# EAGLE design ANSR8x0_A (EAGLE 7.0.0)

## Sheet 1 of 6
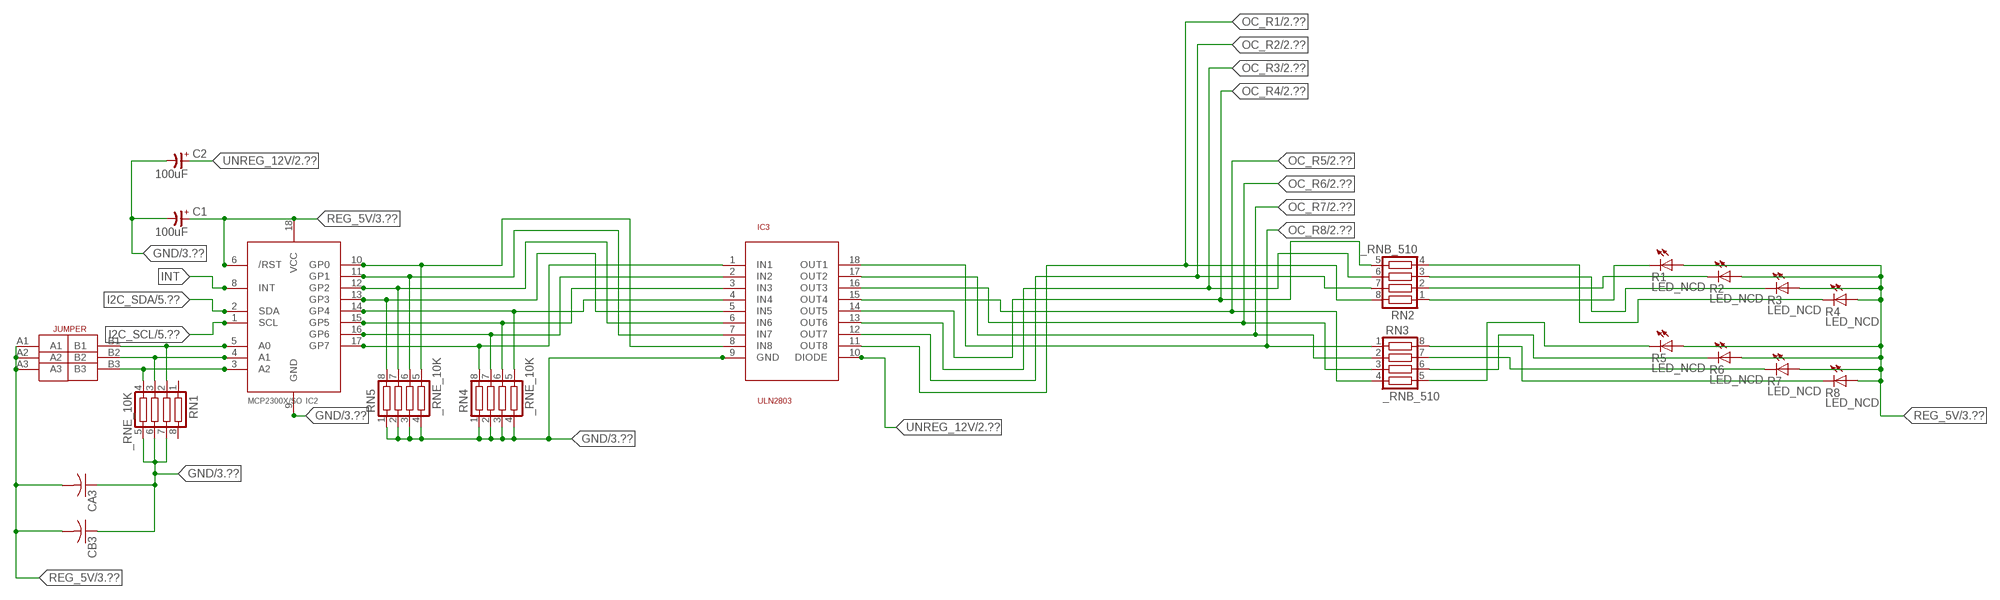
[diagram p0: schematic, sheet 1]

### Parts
C1  100uF  CP-E-025X060  [E-025X060]
C2  100uF  CP-E-025X060  [E-025X060]
CA3  CC1206KRX7R9BB104C1206K  [CC1206KRX7R9BB104]
CB3  TMK316F106ZL-TC1206K  [TMK316F106ZL-T]
IC2  MCP2300X/SO  [SO18W]
IC3  ULN2803  [SO18L]
R1  LED_NCD  [CHIPLED_0603]
R2  LED_NCD  [CHIPLED_0603]
R3  LED_NCD  [CHIPLED_0603]
R4  LED_NCD  [CHIPLED_0603]
R5  LED_NCD  [CHIPLED_0603]
R6  LED_NCD  [CHIPLED_0603]
R7  LED_NCD  [CHIPLED_0603]
R8  LED_NCD  [CHIPLED_0603]
RN1  _RNE_10K  [RNE]
RN2  _RNB_510  [RNB]
RN3  _RNB_510  [RNB]
RN4  _RNE_10K  [RNE]
RN5  _RNE_10K  [RNE]
U$18  JUMPER_3X2  [JUMPER_3X2]

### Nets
GND: C1.- C2.- CA3.1 CB3.1 IC2.9(GND) IC3.9(GND) RN1.5 RN1.6 RN1.7 RN4.1 RN4.2 RN4.3 RN4.4 RN5.1 RN5.2 RN5.3 RN5.4 ; also sheet 3,4,5,6
GP4: IC2.14(GP4) IC3.4(IN4) RN4.5
GP6: IC2.16(GP6) IC3.2(IN2) RN4.7
I2C_SCL: IC2.1(SCL) ; also sheet 5,6
I2C_SDA: IC2.2(SDA) ; also sheet 5,6
INT: IC2.8(INT)
N$6: IC2.5(A0) RN1.2 U$18.B1
N$7: IC2.4(A1) RN1.3 U$18.B2
N$8: IC2.3(A2) RN1.4 U$18.B3
N$20: R1.C RN2.1
N$21: IC2.12(GP2) IC3.6(IN6) RN5.7
N$22: IC2.11(GP1) IC3.7(IN7) RN5.6
N$23: IC2.10(GP0) IC3.8(IN8) RN5.5
N$29: R2.C RN2.2
N$30: R3.C RN2.3
N$31: R4.C RN2.4
N$32: R8.C RN3.8
N$81: R7.C RN3.7
N$82: R6.C RN3.6
N$83: R5.C RN3.5
N$89: IC2.13(GP3) IC3.5(IN5) RN5.8
N$93: IC2.15(GP5) IC3.3(IN3) RN4.6
N$94: IC2.17(GP7) IC3.1(IN1) RN4.8
OC_R1: IC3.11(OUT8) RN2.8 ; also sheet 2
OC_R2: IC3.12(OUT7) RN2.7 ; also sheet 2
OC_R3: IC3.13(OUT6) RN2.6 ; also sheet 2
OC_R4: IC3.14(OUT5) RN2.5 ; also sheet 2
OC_R5: IC3.15(OUT4) RN3.4 ; also sheet 2
OC_R6: IC3.16(OUT3) RN3.3 ; also sheet 2
OC_R7: IC3.17(OUT2) RN3.2 ; also sheet 2
OC_R8: IC3.18(OUT1) RN3.1 ; also sheet 2
REG_5V: C1.+ CA3.2 CB3.2 IC2.6(/RST) IC2.18(VCC) R1.A R2.A R3.A R4.A R5.A R6.A R7.A R8.A U$18.A1 U$18.A2 U$18.A3 ; also sheet 3,4,5,6
UNREG_12V: C2.+ IC3.10(DIODE) ; also sheet 2,3
Unconnected: RN1.1 RN1.8

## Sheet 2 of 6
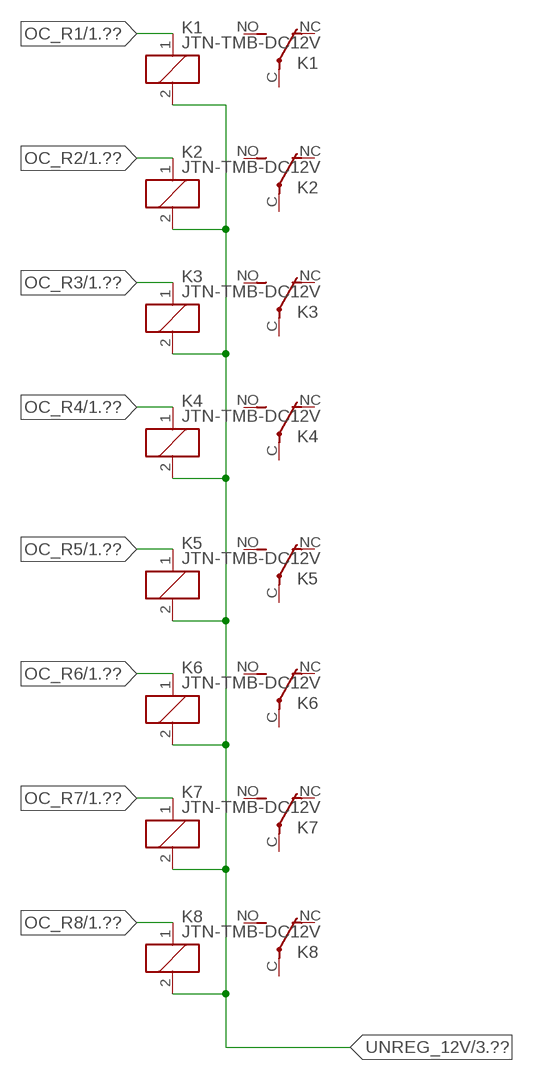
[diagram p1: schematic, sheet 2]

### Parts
K1  JTN-TMB-DC12V  [JT-TMB]
K2  JTN-TMB-DC12V  [JT-TMB]
K3  JTN-TMB-DC12V  [JT-TMB]
K4  JTN-TMB-DC12V  [JT-TMB]
K5  JTN-TMB-DC12V  [JT-TMB]
K6  JTN-TMB-DC12V  [JT-TMB]
K7  JTN-TMB-DC12V  [JT-TMB]
K8  JTN-TMB-DC12V  [JT-TMB]

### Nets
OC_R1: K1.1(C1) ; also sheet 1
OC_R2: K2.1(C1) ; also sheet 1
OC_R3: K3.1(C1) ; also sheet 1
OC_R4: K4.1(C1) ; also sheet 1
OC_R5: K5.1(C1) ; also sheet 1
OC_R6: K6.1(C1) ; also sheet 1
OC_R7: K7.1(C1) ; also sheet 1
OC_R8: K8.1(C1) ; also sheet 1
UNREG_12V: K1.2(C2) K2.2(C2) K3.2(C2) K4.2(C2) K5.2(C2) K6.2(C2) K7.2(C2) K8.2(C2) ; also sheet 1,3
Unconnected: K1.C(COM) K1.NC K1.NO K2.C(COM) K2.NC K2.NO K3.C(COM) K3.NC K3.NO K4.C(COM) K4.NC K4.NO K5.C(COM) K5.NC K5.NO K6.C(COM) K6.NC K6.NO K7.C(COM) K7.NC K7.NO K8.C(COM) K8.NC K8.NO

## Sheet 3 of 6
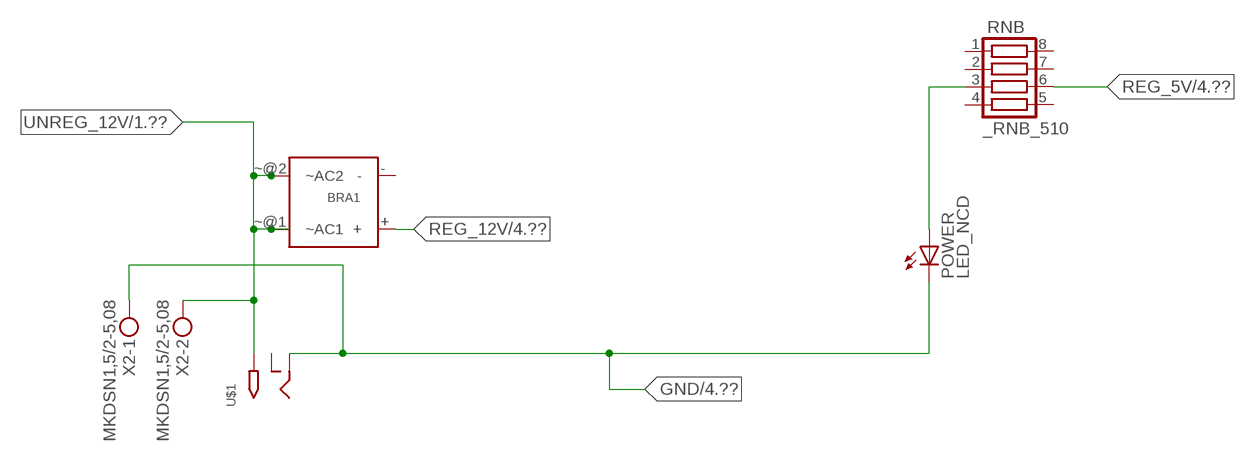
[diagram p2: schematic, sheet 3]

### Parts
BRA1  MB2S_  [MB2S]
POWER  LED_NCD  [CHIPLED_0603]
RNB  _RNB_510  [RNB]
U$1  2.1MMJACK  [PJ-102A]
X2  MKDSN1,5/2-5,08  [MKDSN1,5/2-5,08]

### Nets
GND: POWER.C U$1.RING X2.1 ; also sheet 1,4,5,6
N$2: POWER.A RNB.3
REG_5V: RNB.6 ; also sheet 1,4,5,6
REG_12V: BRA1.+ ; also sheet 4
UNREG_12V: BRA1.~@1(~AC1) BRA1.~@2(~AC2) U$1.TIP X2.2 ; also sheet 1,2
Unconnected: BRA1.- RNB.1 RNB.2 RNB.4 RNB.5 RNB.7 RNB.8 U$1.RING_SW

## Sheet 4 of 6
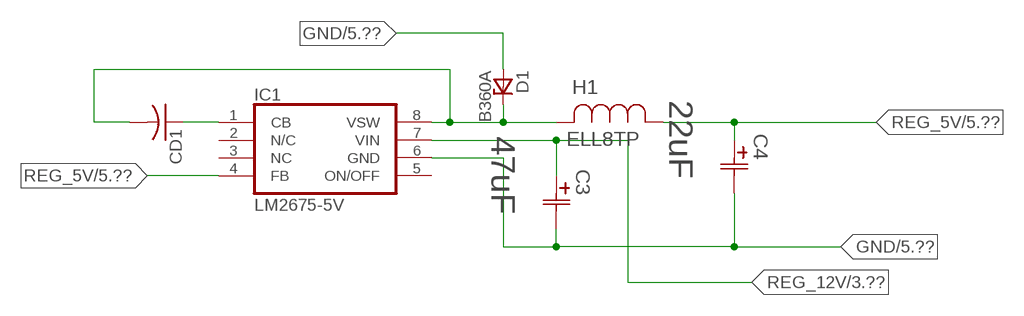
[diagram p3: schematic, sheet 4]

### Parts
C3  47uF  490-5463-6-NDCAP  [C2917(7343)-Y]
C4  22uF  490-5463-6-NDCAP  [C2917(7343)-Y]
CD1  _CD_10NF_50VC1206K  [_CD_10NF_50V]
D1  B360A  [DO214AC_ZENER]
H1  ELL8TP  [IND_ELL8TP]
IC1  LM2675-5V  LM2675  [SO-8]

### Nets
GND: C3.2(C2) C4.2(C2) D1.A IC1.6(GND) ; also sheet 1,3,5,6
N$1: CD1.2 D1.C H1.2 IC1.8(VSW)
N$3: CD1.1 IC1.1(CB)
REG_5V: C4.1(C1) H1.1 IC1.4(FB) ; also sheet 1,3,5,6
REG_12V: C3.1(C1) IC1.7(VIN) ; also sheet 3
Unconnected: IC1.2(N/C) IC1.5(ON/OFF)

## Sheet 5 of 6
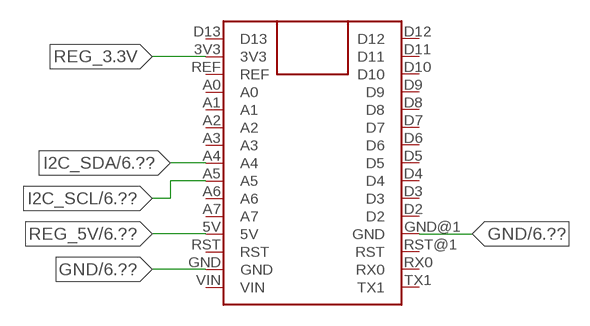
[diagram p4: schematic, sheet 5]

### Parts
FOR_NANO  ARDUINO_NANO  [ARDUINO_NANO]

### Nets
GND: FOR_NANO.GND FOR_NANO.GND@1(GND) ; also sheet 1,3,4,6
I2C_SCL: FOR_NANO.A5 ; also sheet 1,6
I2C_SDA: FOR_NANO.A4 ; also sheet 1,6
REG_3.3V: FOR_NANO.3V3
REG_5V: FOR_NANO.5V ; also sheet 1,3,4,6
Unconnected: FOR_NANO.A0 FOR_NANO.A1 FOR_NANO.A2 FOR_NANO.A3 FOR_NANO.A6 FOR_NANO.A7 FOR_NANO.D2 FOR_NANO.D3 FOR_NANO.D4 FOR_NANO.D5 FOR_NANO.D6 FOR_NANO.D7 FOR_NANO.D8 FOR_NANO.D9 FOR_NANO.D10 FOR_NANO.D11 FOR_NANO.D12 FOR_NANO.D13 FOR_NANO.REF FOR_NANO.RST FOR_NANO.RST@1(RST) FOR_NANO.RX0 FOR_NANO.TX1 FOR_NANO.VIN

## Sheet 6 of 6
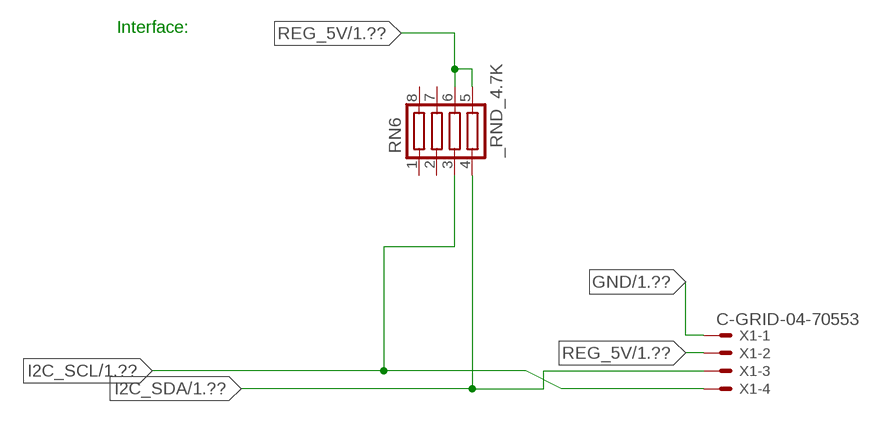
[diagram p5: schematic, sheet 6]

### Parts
RN6  _RND_4.7K  [RND]
X1  C-GRID-04-70553  [70553-04]

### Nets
GND: X1.1 ; also sheet 1,3,4,5
I2C_SCL: RN6.3 X1.4 ; also sheet 1,5
I2C_SDA: RN6.4 X1.3 ; also sheet 1,5
REG_5V: RN6.5 RN6.6 X1.2 ; also sheet 1,3,4,5
Unconnected: RN6.1 RN6.2 RN6.7 RN6.8

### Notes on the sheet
- Interface:

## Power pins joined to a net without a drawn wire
NC: IC1.3(NC)

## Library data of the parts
BRA1 = NCD_ULTIMATE_LIBRARY:MB2S: Bridge Rectifier BRA MB2S 200V 500ma Digikey MB2S-TPMSTR-ND/MB2S-TP
C1 C2 = NCD_ULTIMATE_LIBRARY:CP-: Capacitors All Kinds POLARIZED CAP
C3 C4 = NCD_ULTIMATE_bhaskar:490-5463-6-ND: NCD CAP
CA3 = NCD_ULTIMATE_LIBRARY:CC1206KRX7R9BB104: Capacitor CA .1uF 50V SMT C1206K CC1206KRX7R9BB104
CB3 = NCD_ULTIMATE_LIBRARY:TMK316F106ZL-T: Capacitor CB 10uF SMT 1206 TMK316F106ZL-T
CD1 = NCD_ULTIMATE_LIBRARY:_CD_10NF_50V: Capacitor 10nF SMT
D1 = NCD_ULTIMATE_bhaskar:B360A: NCD DIODE B350A/B360A
FOR_NANO = NCD_ULTIMATE_CONNECTORS:ARDUINO_NANO
H1 = NCD_ULTIMATE_bhaskar:ELL8TP: NCD coil
IC1 = NCD_ULTIMATE_bhaskar:LM2675: LM2675 NCD http://www.ti.com/lit/ds/symlink/lm2675.pdf
IC2 = NCD_ULTIMATE_LIBRARY:MCP2300X: Semiconductor Port Expander I/O 8-Bit I2C MCP23008 Inexpensive i2c i/o expander - 8 general purpose i/o pins with optional pullups
IC3 = NCD_ULTIMATE_LIBRARY:ULN2803: Semiconductor 8 O.C. N-Channel Transistor Driver Digikey ULN2803AFWGCELTR-ND/ULN2803AFWG,C,EL
K1-K8 = NCD_ULTIMATE_LIBRARY:JT?-*: RELAY COMPACT ECONOMICAL 30 AMP. RELAY NAiS Source: http://www.mew-europe.com/.. en_ds_61212_0000.pdf
POWER = NCD_ULTIMATE_bhaskar:LED_NCD
R1-R8 = NCD_ULTIMATE_LIBRARY:LED_NCD: LED Digikey 754-1132-2-ND/APT2012SRCPRV
RN1 RN4 RN5 = NCD_ULTIMATE_LIBRARY:_RNE_10K: Resistor Array RNE SMT 10K x 4 Single Resistor Source: http://www.ctscorp.com/components/Datasheets/CTSChipArrayDs.pdf Digikey 742C083103JPTR-ND/742C083103JP; OC_FARNELL: unknown; OC_NEWARK: unknown
RN2 RN3 RNB = NCD_ULTIMATE_LIBRARY:_RNB_510: Resistor Array RNB SMT 510 x 4 Single Resistor Source: http://www.ctscorp.com/components/Datasheets/CTSChipArrayDs.pdf Digikey 742C083511JPTR-ND/ 742C083511JP; OC_FARNELL: unknown; OC_NEWARK: unknown
RN6 = NCD_ULTIMATE_LIBRARY:_RND_4.7K: Resistor Array RND SMT 4.7K x 4 Single Resistor Source: http://www.ctscorp.com/components/Datasheets/CTSChipArrayDs.pdf Digikey 742C083472JPTR-ND/742C083472JP; OC_FARNELL: unknown; OC_NEWARK: unknown
U$1 = NCD_ULTIMATE_CONNECTORS:2.1MMJACK: 2.1mm x 5.5mm DC jack with internal switch. Digikey part #PJ-102A, 4UCON part #05537 By microbuilder.eu
U$18 = NCD_ULTIMATE_CONNECTORS:JUMPER_3X2
X1 = NCD_ULTIMATE_CONNECTORS:C-GRID-04: CONNECTOR 4-Pos I2C wire to board 2.54 mm (0.100") pitch header Digikey WM1342-ND/0015912045; OC_FARNELL: unknown; OC_NEWARK: unknown
X2 = NCD_ULTIMATE_CONNECTORS:MKDSN1,5/2-5,08: MKDSN 1,5/ 2-5,08 Printklemme

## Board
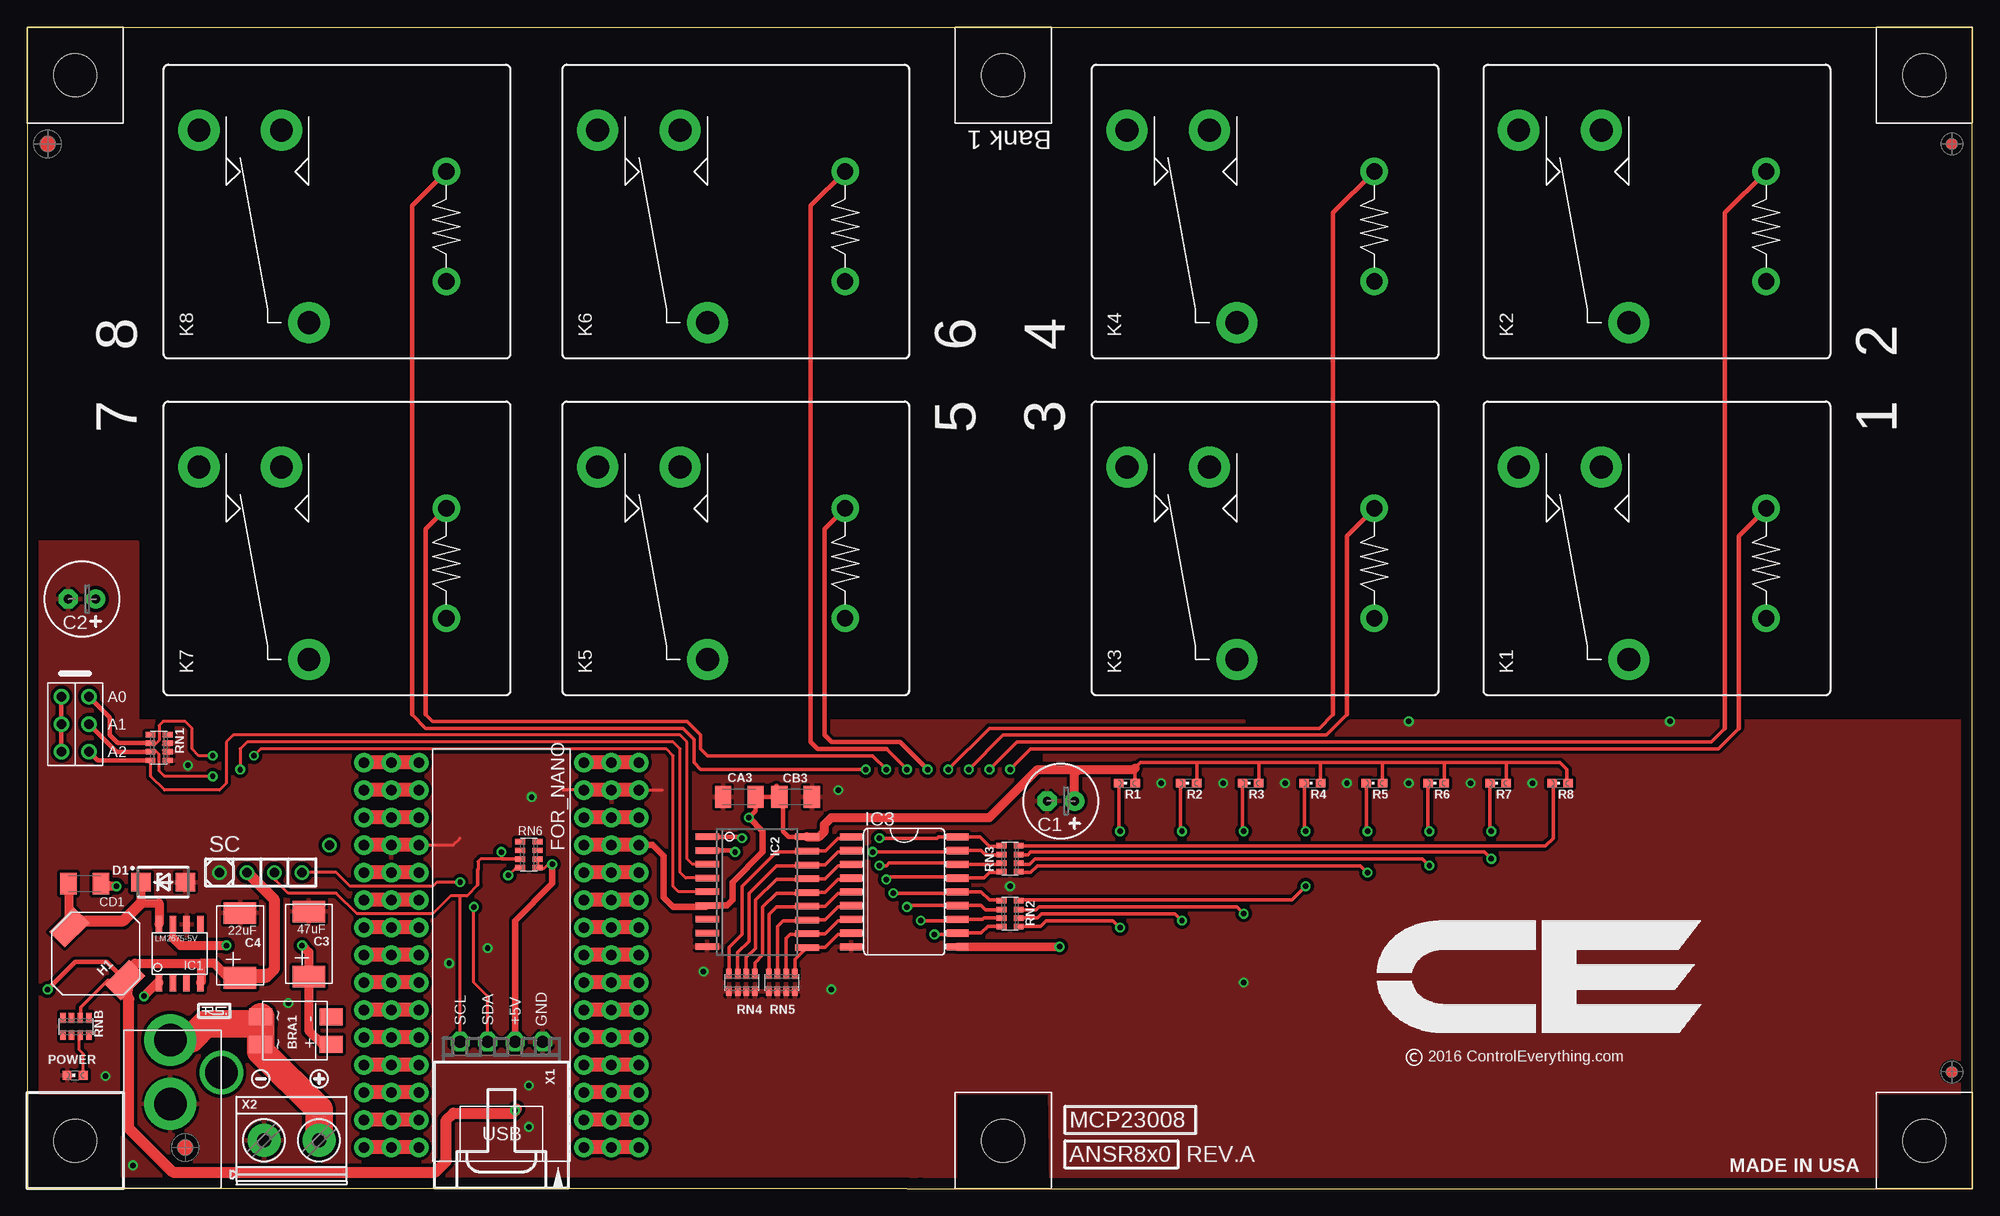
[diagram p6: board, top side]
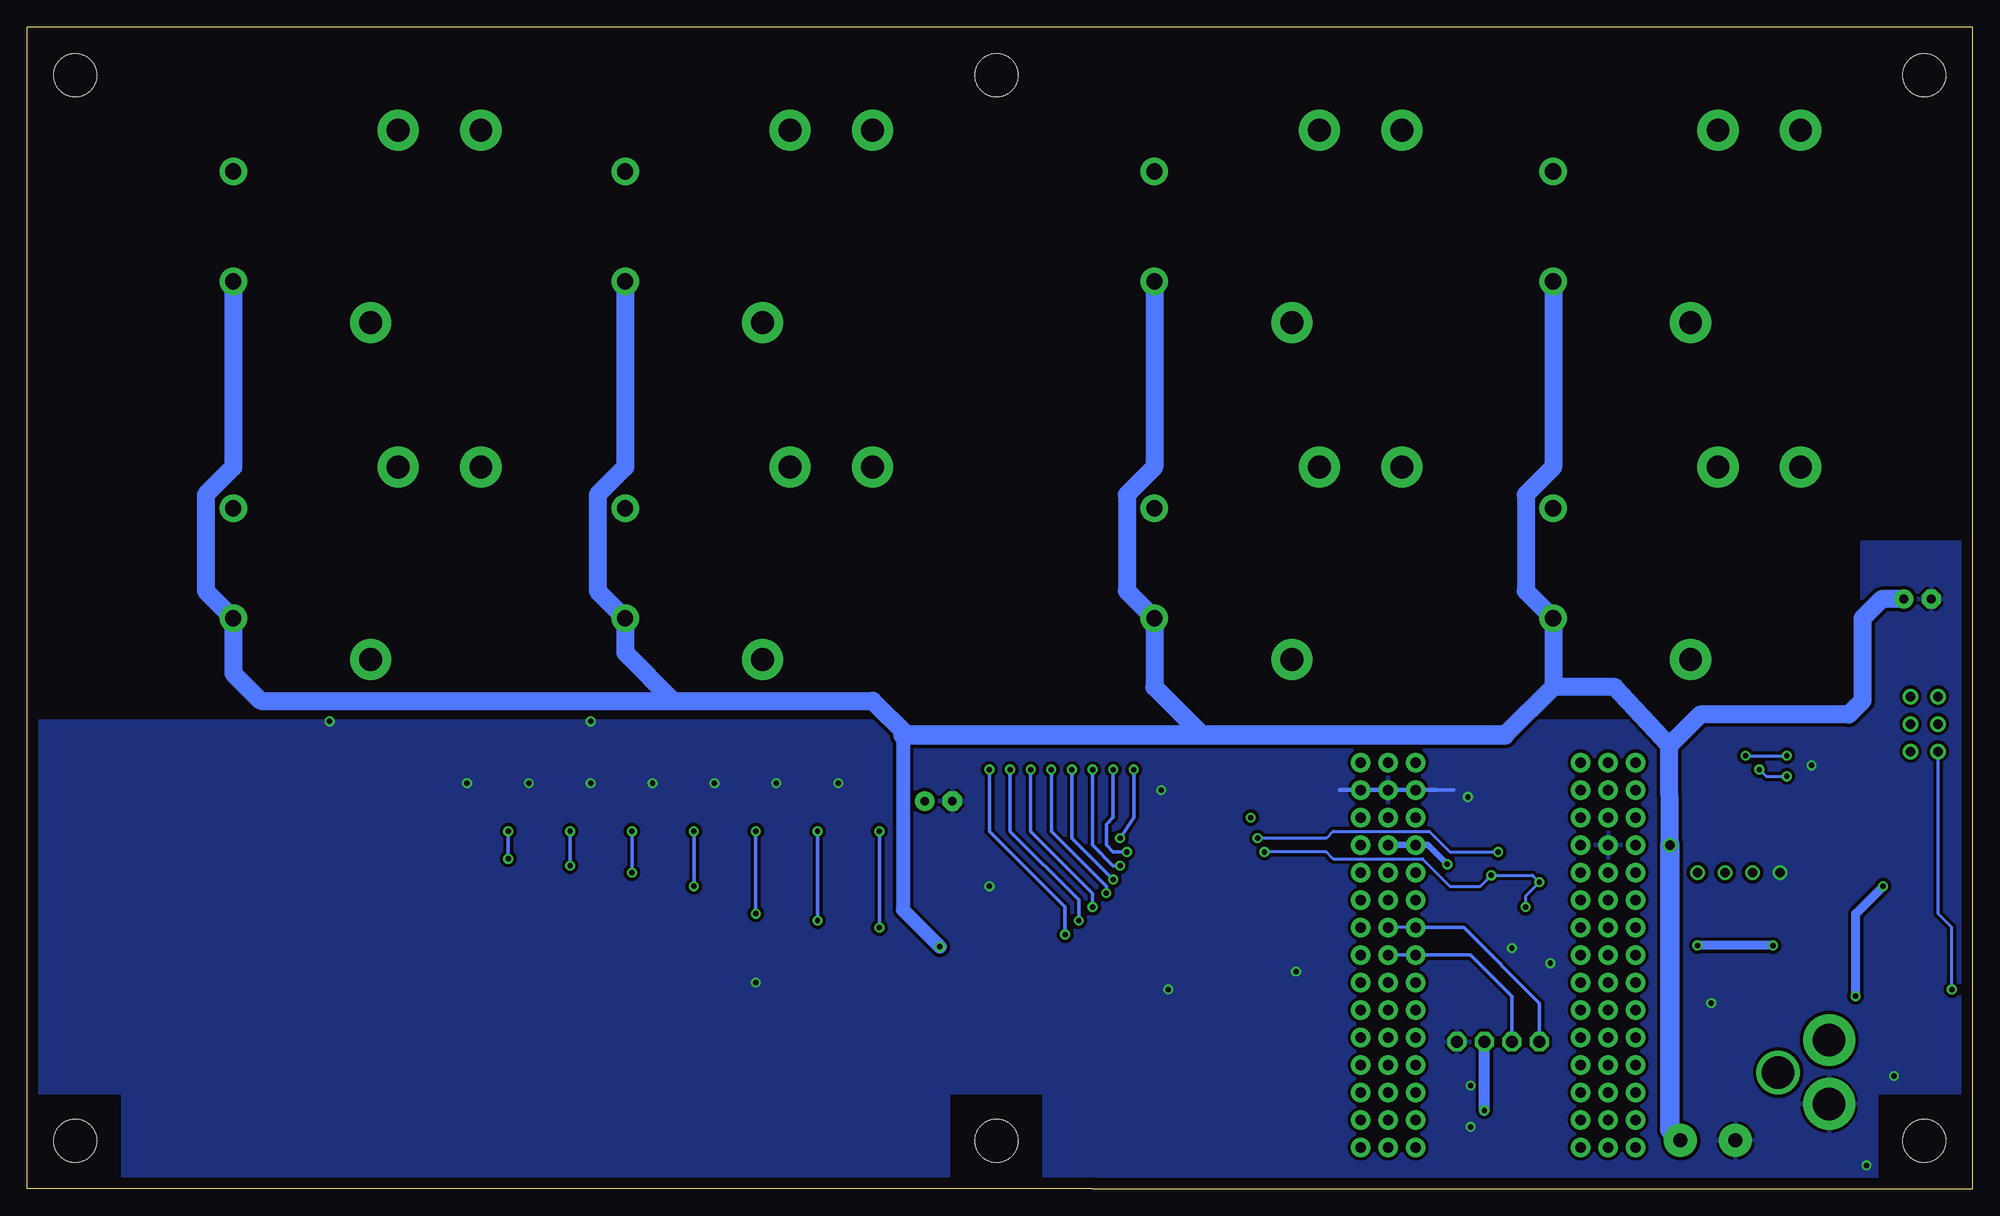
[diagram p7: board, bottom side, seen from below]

Size 179.71 x 107.33 mm. Coordinates in mm from the lower left corner, seen from the top.
Outline: 81.28,0 82.53,0
Outline: 0,65.71 0,64.77
Outline: 0,64.77 0,0 81.28,0
Outline: 81.28,0 179.71,0 179.71,107.31
Outline: 0,107.31 0,64.77
Outline: 0.02,107.33 179.71,107.33
Copper layers (1*16): Top 0.035mm / dielectric 1.5mm / Bottom 0.035mm
Design rules "default": minimum track width 10mil, minimum drill 24mil, track to track 8mil, track to pad 8mil, pad to pad 8mil, via to via 8mil, smd to smd 8mil, copper to edge 40mil, drill to drill 8mil, minimum pad ring 10mil, minimum via ring 8mil, stop-mask expansion 4mil, vias tented up to drill 0mil, thermal gap 10mil
Holes 3.96 mm at 4.45,4.45 4.45,4.45 4.45,4.45 4.45,4.45

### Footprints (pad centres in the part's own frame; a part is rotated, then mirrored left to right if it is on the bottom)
MB2S = smd 1.55 x 2.1: + 0,-6.5; - 2.54,-6.5; ~@1 0,0; ~@2 2.54,0
E-025X060 = drill 0.813 pad 1.778: + -1.27,0 | drill 0.813 pad 1.778 octagon: - 1.27,0
C2917(7343)-Y = smd 2 x 3: 1 -3,0; 2 3,0
CC1206KRX7R9BB104 = smd 1.5 x 2: 1 -1.5,0; 2 1.5,0
TMK316F106ZL-T = smd 1.5 x 2: 1 -1.5,0; 2 1.5,0
_CD_10NF_50V = smd 1.5 x 2: 1 -1.5,0; 2 1.5,0
DO214AC_ZENER = smd 1.8 x 1.7: A 2.05,0; C -2.05,0
ARDUINO_NANO = drill 1 pad 1.778: 3V1 -2.54,-2.54; 3V3 0,-2.54; 5V 0,-27.94; 5V1 -2.54,-27.94; A0 0,-7.62; A1 0,-10.16; A2 0,-12.7; A3 0,-15.24; A4 0,-17.78; A5 0,-20.32; A6 0,-22.86; A7 0,-25.4; A8 -2.54,-7.62; A9 -2.54,-10.16; A10 -2.54,-12.7; A11 -2.54,-15.24; A12 -2.54,-17.78; A13 -2.54,-20.32; A14 -2.54,-22.86; A15 -2.54,-25.4; D1 -2.54,0; D2 20.32,-25.4; D3 20.32,-22.86; D4 20.32,-20.32; D5 20.32,-17.78; D6 20.32,-15.24; D7 20.32,-12.7; D8 20.32,-10.16; D9 20.32,-7.62; D10 20.32,-5.08; D11 20.32,-2.54; D12 20.32,0; D13 0,0; D14 22.86,0; D15 22.86,-2.54; D16 22.86,-5.08; D17 22.86,-7.62; D18 22.86,-10.16; D19 22.86,-12.7; D20 22.86,-15.24; D21 22.86,-17.78; D22 22.86,-20.32; D23 22.86,-22.86; D24 22.86,-25.4; GND 0,-33.02; GND1 -2.54,-33.02; GND@1 20.32,-27.94; GND@2 22.86,-27.94; P$16 2.54,0; P$17 2.54,-2.54; P$18 2.54,-5.08; P$19 2.54,-7.62; P$20 2.54,-10.16; P$21 2.54,-12.7; P$22 2.54,-15.24; P$23 2.54,-17.78; P$24 2.54,-20.32; P$25 2.54,-22.86; P$26 2.54,-25.4; P$27 2.54,-27.94; P$28 2.54,-30.48; P$29 2.54,-33.02; P$30 2.54,-35.56; P$31 17.78,0; P$32 17.78,-2.54; P$33 17.78,-5.08; P$34 17.78,-7.62; P$35 17.78,-10.16; P$36 17.78,-12.7; P$37 17.78,-15.24; P$38 17.78,-17.78; P$39 17.78,-20.32; P$40 17.78,-22.86; P$41 17.78,-25.4; P$42 17.78,-27.94; P$43 17.78,-30.48; P$44 17.78,-33.02; P$45 17.78,-35.56; REF 0,-5.08; REF1 -2.54,-5.08; RST 0,-30.48; RST1 -2.54,-30.48; RST@1 20.32,-30.48; RST@2 22.86,-30.48; RX0 20.32,-33.02; RX1 22.86,-33.02; TX1 20.32,-35.56; TX2 22.86,-35.56; VIN 0,-35.56; VIN1 -2.54,-35.56
IND_ELL8TP = smd 2.054 x 3.2 rotated 45: 1 -2.442,-2.696; 2 2.442,2.442
SO-8 = smd 0.6 x 1.55: 1 -1.905,-2.69; 2 -0.635,-2.69; 3 0.635,-2.69; 4 1.905,-2.69; 5 1.905,2.71; 6 0.635,2.71; 7 -0.635,2.71; 8 -1.905,2.71
SO18W = smd 0.6 x 2.2: 1 -4.445,-4.6; 2 -3.175,-4.6; 3 -1.905,-4.6; 4 -0.635,-4.6; 5 0.635,-4.6; 6 1.905,-4.6; 7 3.175,-4.6; 8 4.445,-4.6; 9 5.715,-4.6; 10 5.775,4.6; 11 4.505,4.6; 12 3.235,4.6; 13 1.965,4.6; 14 0.695,4.6; 15 -0.575,4.6; 16 -1.845,4.6; 17 -3.145,4.6; 18 -4.445,4.6
SO18L = smd 0.66 x 2.032: 1 -5.08,-4.902; 2 -3.81,-4.902; 3 -2.54,-4.902; 4 -1.27,-4.902; 5 0,-4.902; 6 1.27,-4.902; 7 2.54,-4.902; 8 3.81,-4.902; 9 5.08,-4.902; 10 5.08,4.902; 11 3.81,4.902; 12 2.54,4.902; 13 1.27,4.902; 14 0,4.902; 15 -1.27,4.902; 16 -2.54,4.902; 17 -3.81,4.902; 18 -5.08,4.902
JT-TMB = drill 1.5 pad 2.54: 1 5.08,0; 2 -5.08,0 | drill 2.1 pad 3.81: C -8.89,12.7; NC 8.89,22.86; NO 8.89,15.24
CHIPLED_0603 = smd 0.8 x 0.8: A 0,-0.75; C 0,0.75
CHIPLED_0603' = smd 0.8 x 0.876: A 0,-0.75; C 0,0.75
RNE = smd 0.5 x 0.9: 1 -1.2,-0.8; 2 -0.4,-0.8; 3 0.4,-0.8; 4 1.2,-0.8; 5 1.2,0.8; 6 0.4,0.8; 7 -0.4,0.8; 8 -1.2,0.8
RNB = smd 0.5 x 0.9: 1 -1.2,-0.8; 2 -0.4,-0.8; 3 0.4,-0.8; 4 1.2,-0.8; 5 1.2,0.8; 6 0.4,0.8; 7 -0.4,0.8; 8 -1.2,0.8
RND = smd 0.5 x 0.9: 1 -1.2,-0.8; 2 -0.4,-0.8; 3 0.4,-0.8; 4 1.2,-0.8; 5 1.2,0.8; 6 0.4,0.8; 7 -0.4,0.8; 8 -1.2,0.8
PJ-102A = drill 3 pad 4.8: RING 0.1,-3.39; TIP 0.1,-9.29 | drill 3 pad 3.251: RING_SW -4.6,-6.29
PCB_MOUNTING_HOLE = hole 3.962: 4.445,4.445
JUMPER_3X2 = drill 0.9: A1 0,5.08; A2 0,2.54; A3 0,0; B1 2.54,5.08; B2 2.54,2.54; B3 2.54,0
70553-04 = drill 1.1 pad 1.778 octagon: 1 -3.81,-7.62; 2 -1.27,-7.62; 3 1.27,-7.62; 4 3.81,-7.62
MKDSN1,5/2-5,08 = drill 1.3 pad 3.048: 1 -2.561,0.025; 2 2.519,0.025

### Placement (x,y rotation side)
BRA1  21.59,13.34 90 top
C1  95.5,35.81 180 top
C2  5.08,54.48 180 top
C3  26.04,22.61 90 top
C4  19.68,22.48 90 top
CA3  65.79,36.2 0 top
CB3  70.99,36.2 180 top
CD1  5.33,28.19 180 top
D1  12.57,28.32 0 top
FOR_NANO  53.98,3.81 180 top
H1  6.35,21.72 90 top
IC1  14.1,21.72 0 top
IC2  67.44,28.07 270 top
IC3  81.03,27.43 270 top
K1  160.66,57.79 90 top
K2  160.66,88.9 90 top
K3  124.46,57.79 90 top
K4  124.46,88.9 90 top
K5  75.56,57.79 90 top
K6  75.56,88.9 90 top
K7  38.73,57.79 90 top
K8  38.73,88.9 90 top
POWER  4.45,10.48 90 top
R1  LED_NCD  [CHIPLED_0603']  101.6,37.47 90 top
R2  LED_NCD  [CHIPLED_0603']  107.31,37.47 90 top
R3  LED_NCD  [CHIPLED_0603']  113.03,37.47 90 top
R4  LED_NCD  [CHIPLED_0603']  118.75,37.47 90 top
R5  LED_NCD  [CHIPLED_0603']  124.46,37.47 90 top
R6  LED_NCD  [CHIPLED_0603']  130.18,37.47 90 top
R7  LED_NCD  [CHIPLED_0603']  135.89,37.47 90 top
R8  LED_NCD  [CHIPLED_0603']  141.6,37.47 90 top
RN1  12.19,40.77 270 top
RN2  90.81,25.4 90 top
RN3  90.81,30.48 270 top
RN4  66.04,19.05 0 top
RN5  69.72,19.05 0 top
RN6  46.35,30.86 270 top
RNB  4.51,14.99 0 top
U$1  13.34,4.45 180 top
U$2  [VISION_REF15]  14.61,3.81 0 top
U$3  [ICON_MINUS]  21.59,10.16 180 top
U$4  [VISION_REF10]  177.8,10.79 270 top
U$5  [ICON_PLUS]  26.99,10.16 90 top
U$6  PCB_MOUNTING_HOLE  [PCB_MOUNTING_HOLE]  94.61,0 90 top
U$11  PCB_MOUNTING_HOLE  [PCB_MOUNTING_HOLE]  179.71,0 90 top
U$13  [VISION_REF10]  177.8,96.52 270 top
U$14  [VISION_REF15]  1.91,96.52 270 top
U$17  PCB_MOUNTING_HOLE  [PCB_MOUNTING_HOLE]  94.61,98.42 90 top
U$18  3.17,40.39 0 top
U$19  PCB_MOUNTING_HOLE  [PCB_MOUNTING_HOLE]  94.61,98.42 90 top
U$20  PCB_MOUNTING_HOLE  [PCB_MOUNTING_HOLE]  179.71,98.42 90 top
U$21  [ICON_USA]  157.23,1.52 0 top
U$25  PCB_MOUNTING_HOLE  [PCB_MOUNTING_HOLE]  179.71,98.42 90 top
U$31  PCB_MOUNTING_HOLE  [PCB_MOUNTING_HOLE]  8.89,98.42 90 top
U$32  PCB_MOUNTING_HOLE  [PCB_MOUNTING_HOLE]  8.89,98.42 90 top
X1  43.81,5.97 180 top
X2  24.45,4.45 0 top

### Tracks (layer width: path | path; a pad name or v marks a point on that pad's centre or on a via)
GND  (via drill 0.5, 0.9)
  Top 0.254: 36.2,31.75 39.37,31.75 40.01,32.39 | FOR_NANO.GND@1 32.38,31.75 | 49.53,36.83 56.52,36.83 58.67,36.83
  Top 1.016: X1.1 47.62,13.74
  Bottom 0.254: 51.44,36.83 FOR_NANO.GND
  Bottom 0.305: 47.88,36.83 49.53,36.83 51.44,36.83
  Bottom 0.406: 49.53,36.83 58.42,36.83
  other vias: 14.86,39.12 62.48,20.07 127.64,37.47 112.39,19.05 133.35,37.47 139.06,37.47 121.92,37.47 116.2,37.47 110.49,37.47 104.78,37.47 90.81,27.94 127.64,43.18 151.76,43.18 74.3,18.41 74.93,36.83 9.78,2.16 17.78,29.21 46.35,9.53 46.61,36.2 46.35,5.72 42.55,22.23 38.99,20.83 7.24,10.41 24.13,17.15
  pour Bottom (isolate 0.305): -3.17,8.89 8.89,8.89 8.89,0 85.72,0 85.72,8.89 112.39,8.89 112.39,43.18 10.16,43.18 10.16,59.69 -3.17,59.69
  pour Top (isolate 0.305): -1.27,8.89 8.89,8.89 8.89,0 85.72,0 85.72,8.89 112.39,8.89 112.39,43.18 10.16,43.18 10.16,59.69 -1.27,59.69
  pour Top (isolate 0.305): 112.39,43.18 180.97,43.18 181.61,8.89 170.81,8.89 170.81,0 111.76,0
  pour Bottom (isolate 0.305): 94.61,0 94.61,43.18 182.25,43.18 182.88,8.89 170.81,8.89 170.81,0
  pour Top (isolate 0.305): 185.42,8.89 170.81,8.89 170.81,0 94.61,0 93.98,43.18 184.78,43.18
  pour Top (isolate 0.305): 170.81,8.89 170.81,0 94.61,0 93.98,43.18 186.69,43.18 187.32,8.89
GP4
  Top 0.305: RN4.5 67.24,20.88 67.94,21.59 67.94,26.04 69.22,27.3 71.97,27.3 IC2.14 73.73,27.37 74.93,28.57 76,28.57 IC3.4
GP6
  Top 0.305: RN4.7 65.64,21.83 66.67,22.86 66.67,27.3 69.22,29.84 71.97,29.84 IC2.16 73.73,29.91 74.93,31.12 76,31.12 IC3.2
I2C_SCL  (via drill 0.5, 0.9)
  Top 0.254: 41.64,28.05 40.64,27.05 40.01,27.05 | 40.01,27.05 39.12,27.05 37.47,25.4 30.48,25.4 28.57,27.3 24.13,27.3 22.86,28.57 v22.86,29.21 | X1.4 40.01,27.05 | v43.81,31.12 43.81,30.48 45.54,30.48 RN6.3 41.89,30.46 41.66,30.23 41.66,29.5
  Top 0.305: 41.64,28.05 41.64,29.48 41.66,29.5
  Top 0.406: IC2.1 65.91,32.51 v66.04,32.39
  Bottom 0.254: v43.81,31.12 48.26,31.12 50.16,33.02 59.05,33.02 59.69,32.39 v66.04,32.39 | 51.44,24.13 FOR_NANO.A5
  Bottom 0.305: 51.44,24.13 46.99,24.13 40.01,17.15 X1.4
I2C_SDA  (via drill 0.5, 0.9)
  Top 0.254: RN6.4 45.16,29.66 v44.45,28.96 | 40,28.33 v40.01,28.32 37.85,28.32 37.47,27.94 29.84,27.94 28.57,29.21 v25.4,29.21 | X1.3 42.55,17.78 41.27,19.05 v41.27,26.04
  Top 0.406: IC2.2 65.28,31.24 v65.41,31.12
  Bottom 0.254: v41.27,26.04 41.27,27.05 v40.01,28.32 40.64,28.96 v44.45,28.96 45.47,27.94 48.26,27.94 50.8,30.48 59.05,30.48 59.69,31.12 v65.41,31.12
  Bottom 0.305: FOR_NANO.A4 46.35,21.59 42.55,17.78 X1.3
N$1
  Top 0.813: H1.2 3.88,24.77 | D1.C 10.52,26.4 12.19,26.38 IC1.8 | CD1.2 3.83,24.15 4.45,24.77
  Top 1.016: 3.88,24.77 4.45,24.77 8.89,24.77 10.52,26.4
N$2
  Top 0.254: POWER.A 5.2,12.46 4.83,12.83 4.83,14.1 RNB.3
  Top 0.406: 4.95,14.14 RNB.3
N$3  (via drill 0.5)
  Top 0.813: IC1.1 12.04,19.03 v10.79,17.78 | v8.26,27.94 7.72,27.94 CD1.1
  Bottom 0.813: v10.79,17.78 10.79,25.4 v8.26,27.94
N$6  (via drill 0.5)
  Top 0.254: IC2.5 60.2,27.43 59.69,27.94 59.69,40 59.05,40.64 21.59,40.64 v20.95,40 | v17.14,40 15.88,40 15.24,40.64 15.24,42.55 14.61,43.18 12.57,43.18 12.19,42.8 12.19,41.4 11.94,41.15 11.41,41.15 RN1.2
  Top 0.406: RN1.2 8.36,41.17 7.62,41.91 7.62,43.56 U$18.B1
  Bottom 0.254: v20.95,40 v17.14,40
N$7  (via drill 0.5)
  Top 0.254: IC2.4 60.83,28.7 60.33,29.21 60.33,40.64 59.69,41.27 20.32,41.27 19.68,40.64 v19.68,38.73 | v17.14,38.1 12.7,38.1 12.19,38.61 12.19,40.13 11.94,40.39 11.41,40.39 RN1.3
  Top 0.406: RN1.3 8.27,40.37 U$18.B2
  Bottom 0.254: v19.68,38.73 19.05,38.1 v17.14,38.1
N$8
  Top 0.254: IC2.3 61.47,29.97 60.96,30.48 60.96,41.27 60.33,41.91 19.05,41.91 18.41,41.27 18.41,37.47 17.78,36.83 12.7,36.83 11.43,38.1 11.43,39.53 RN1.4
  Top 0.406: RN1.4 6.53,39.57 U$18.B3
N$20  (via drill 0.5)
  Top 0.305: R1.C 100.85,33.14 v100.97,33.02 | v100.97,24.13 100.33,24.77 94.11,24.77 93.6,24.26 91.66,24.26 RN2.1
  Bottom 0.305: v100.97,33.02 v100.97,24.13
N$21
  Top 0.305: RN5.7 69.32,24.24 69.85,24.77 71.97,24.77 IC2.12 73.73,24.83 74.93,26.04 76,26.04 IC3.6
N$22
  Top 0.305: RN5.6 70.12,23.13 70.48,23.5 71.97,23.5 IC2.11 73.73,23.56 74.93,24.77 76,24.77 IC3.7
N$23
  Top 0.254: 71.97,22.23 IC2.10
  Top 0.305: RN5.5 70.92,21.18 IC2.10 73.73,22.29 74.93,23.5 76,23.5 IC3.8
N$29  (via drill 0.5)
  Top 0.305: R2.C 106.56,33.14 v106.68,33.02 | v106.68,24.77 106.05,25.4 93.73,25.4 93.34,25.02 91.62,25.02 RN2.2
  Bottom 0.305: v106.68,33.02 v106.68,24.77
N$30  (via drill 0.5)
  Top 0.305: R3.C 112.28,33.14 v112.39,33.02 | v112.39,25.4 111.76,26.04 93.47,26.04 93.22,25.78 91.62,25.78 RN2.3
  Bottom 0.305: v112.39,33.02 v112.39,25.4
N$31  (via drill 0.5)
  Top 0.305: R4.C 118,33.14 v118.11,33.02 | v118.11,27.94 116.84,26.67 91.67,26.67 RN2.4
  Bottom 0.305: v118.11,33.02 v118.11,27.94
N$32
  Top 0.305: RN3.8 140.26,31.68 140.97,32.39 140.97,37.35 R8.C
N$81  (via drill 0.5)
  Top 0.305: R7.C 135.14,33.14 v135.25,33.02 | v135.25,30.48 134.62,31.12 92.71,31.12 92.46,30.86 91.62,30.86 RN3.7
  Bottom 0.305: v135.25,33.02 v135.25,30.48
N$82  (via drill 0.5)
  Top 0.305: R6.C 129.43,33.14 v129.54,33.02 | v129.54,29.84 128.91,30.48 93.09,30.48 92.58,29.97 91.71,29.97 RN3.6
  Bottom 0.305: v129.54,33.02 v129.54,29.84
N$83  (via drill 0.5)
  Top 0.305: R5.C 123.71,33.14 v123.83,33.02 | v123.83,29.21 123.19,29.84 93.34,29.84 92.71,29.21 91.67,29.21 RN3.5
  Bottom 0.305: v123.83,33.02 v123.83,29.21
N$89
  Top 0.305: RN5.8 68.52,25.34 69.22,26.04 71.97,26.04 IC2.13 73.73,26.1 74.93,27.3 76,27.3 IC3.5
N$93
  Top 0.305: RN4.6 66.44,21.36 67.31,22.23 67.31,26.67 69.22,28.57 71.97,28.57 IC2.15 73.73,28.64 74.93,29.84 76,29.84 IC3.3
N$94
  Top 0.305: RN4.8 64.84,22.3 66.04,23.5 66.04,27.94 69.22,31.12 71.94,31.12 IC2.17 73.76,31.21 74.93,32.39 76,32.39 IC3.1
OC_R1  (via drill 0.5)
  Top 0.305: RN2.8 89.95,24.26 88.77,24.26 88.14,23.62 IC3.11 85.8,23.5 v83.82,23.5 | v90.81,38.73 92.71,40.64 156.21,40.64 158.12,42.55
  Top 0.406: K1.1 158.12,60.33 158.12,42.55
  Bottom 0.305: v90.81,38.73 90.81,33.02 83.82,26.04 v83.82,23.5
OC_R2  (via drill 0.5)
  Top 0.305: RN2.7 89.99,25.02 88.39,25.02 88.27,24.89 IC3.12 85.8,24.77 v82.55,24.77 | v88.9,38.73 91.44,41.27 155.57,41.27 156.84,42.55
  Top 0.406: K2.1 156.84,90.17 156.84,42.55
  Bottom 0.305: v88.9,38.73 88.9,33.02 82.55,26.67 v82.55,24.77
OC_R3  (via drill 0.5)
  Top 0.305: RN2.6 89.99,25.78 88.52,25.78 88.14,26.16 IC3.13 81.53,26.16 81.41,26.04 v81.28,26.04 | 121.92,43.81 120.02,41.91 90.17,41.91 v87,38.73
  Top 0.406: K3.1 121.92,60.33 121.92,43.81
  Bottom 0.305: v87,38.73 87,33.02 81.28,27.3 v81.28,26.04
OC_R4  (via drill 0.5)
  Top 0.305: RN2.5 89.94,26.67 88.9,26.67 88.14,27.43 IC3.14 85.8,27.3 v80.01,27.3 | 120.65,43.81 119.38,42.55 88.9,42.55 v85.09,38.73
  Top 0.406: K4.1 120.65,90.17 120.65,43.81
  Bottom 0.305: v85.09,38.73 85.09,33.02 80.01,27.94 v80.01,27.3
OC_R5  (via drill 0.5)
  Top 0.305: RN3.4 89.94,29.21 88.9,29.21 88.39,28.7 IC3.15 85.8,28.83 79.63,28.83 v79.38,28.57
  Top 0.406: K5.1 73.66,60.96 73.66,41.91 74.3,41.27 80.64,41.27 v83.19,38.73
  Bottom 0.305: v83.19,38.73 83.19,32.39 v79.38,28.57
OC_R6  (via drill 0.5)
  Top 0.305: RN3.3 89.9,29.97 IC3.16 85.8,30.1 79.63,30.1 79.38,29.84 v78.74,29.84 | 79.38,40.64 v81.28,38.73
  Top 0.406: K6.1 72.39,90.81 72.39,41.27 73.03,40.64 79.38,40.64
  Bottom 0.305: v81.28,38.73 81.28,31.75 79.38,29.84 v78.74,29.84
OC_R7  (via drill 0.5)
  Top 0.305: RN3.2 89.99,30.86 88.52,30.86 88.14,31.24 IC3.17 85.8,31.12 v78.11,31.12 | v79.38,38.73 78.11,40 62.87,40 62.23,40.64 62.23,41.91 60.96,43.18 37.47,43.18 36.83,43.81
  Top 0.406: K7.1 36.83,60.96 36.83,43.81
  Bottom 0.305: v79.38,38.73 79.38,34.29 80.01,33.66 80.01,31.75 79.38,31.12 v78.11,31.12
OC_R8  (via drill 0.5)
  Top 0.305: RN3.1 89.95,31.62 88.9,31.62 88.01,32.51 IC3.18 84.2,32.51 84.07,32.39 v78.74,32.39 | v77.47,38.73 62.23,38.73 61.59,39.37 61.59,41.53 60.58,42.55 36.83,42.55 35.56,43.81
  Top 0.406: K8.1 35.56,90.81 35.56,43.81
  Bottom 0.305: v77.47,38.73 77.47,34.29 v78.74,32.39
REG_5V  (via drill 0.5, 0.9)
  Top 0.254: RN6.6 RN6.5 47.23,29.59 47.75,29.59 48.13,29.97 v48.51,29.97
  Top 0.305: R1.A 102.35,38.85 102.87,39.37 107.95,39.37 | 107.95,39.37 113.67,39.37 | 113.67,39.37 119.38,39.37 | 119.38,39.37 125.09,39.37 | 125.09,39.37 130.81,39.37 | 130.81,39.37 136.53,39.37 | 136.53,39.37 141.6,39.37 142.24,38.73 142.24,37.58 R8.A | R7.A 136.64,39.25 136.53,39.37 | R6.A 130.93,39.25 130.81,39.37 | R5.A 125.21,39.25 125.09,39.37 | R4.A 119.5,39.25 119.38,39.37 | R3.A 113.78,39.25 113.67,39.37 | R2.A 108.06,39.25 107.95,39.37 | H1.1 7.46,19.27 4.95,16.76 4.95,15.83 RNB.6
  Top 0.406: U$18.A3 U$18.A2 U$18.A1 | IC2.18 70.36,32.51 69.85,33.02 69.85,36.47 CB3.2 CA3.2 67.29,34.9 v66.67,34.29 | v1.91,18.41 4.45,20.95 7.37,20.95 H1.1
  Top 0.61: 69.22,37.11 CB3.2 | v66.67,34.29 67.94,33.02 67.94,31.12 65.15,28.32 65.15,26.67 64.64,26.16 IC2.6 62.71,26.04 59.69,26.04 58.8,26.92 58.8,30.73 57.78,31.75 FOR_NANO.5V | v48.51,29.97 48.51,28.19 45.09,24.77 X1.2
  Top 0.813: IC2.18 73.15,32.51 73.66,33.02 73.66,33.66 74.3,34.29 88.9,34.29 93.34,38.73 97.16,38.73 | 97.16,38.73 102.23,38.73 102.35,38.85 | C1.+ 96.77,38.35 97.16,38.73 | 16.13,20.83 9.96,20.83 H1.1 | 16.13,20.83 17.27,20.83 18.41,19.69 20.75,19.69 C4.1 | IC1.4 16.13,19.15 16.13,20.83
  Top 1.016: H1.1 9.27,18.41 9.27,17.65 9.4,17.53 9.4,5.59 13.46,1.52 37.72,1.52 38.73,2.54 38.73,6.35 39.37,6.99 44.83,6.99 v45.09,7.24 45.21,7.37 | 22.05,19.69 22.23,19.69 22.86,20.32 22.86,26.67 v20.32,29.21
  Top 1.27: 20.75,19.69 22.05,19.69
  Bottom 0.254: U$18.A3 3.17,25.4 1.91,24.13 v1.91,18.41
  Bottom 0.61: FOR_NANO.5V 50.29,31.75 v48.51,29.97
  Bottom 1.016: v45.09,7.24 X1.2
REG_12V  (via drill 0.5)
  Top 0.61: IC1.7 13.46,23.16 | 14.1,22.48 14.15,22.48
  Top 0.813: v18.41,22.48 14.15,22.48 13.46,23.16 | v25.4,22.48 26.04,21.84 C3.1 26.04,14.61 27.3,13.34 BRA1.+
  Bottom 0.813: v18.41,22.48 v25.4,22.48
UNREG_12V  (via drill 0.5, 0.9)
  Top 0.762: v95.38,22.35 IC3.10
  Top 2.54: X2.2 26.97,7.32 21.59,12.7 BRA1.~@1 21.59,15.24 | 21.59,15.24 BRA1.~@2 | U$1.TIP 15.14,13.87 16.51,15.24 21.59,15.24
  Bottom 1.27: 98.81,41.91 98.81,25.78 v95.38,22.35
  Bottom 1.676: K2.2 160.66,66.67 163.19,64.13 163.19,55.24 K1.2 160.66,47.62 158.12,45.09 120.02,45.09 | K4.2 124.46,66.67 127,64.13 127,55.24 K3.2 124.46,49.53 120.02,45.09 | K6.2 75.56,66.67 78.11,64.13 78.11,55.24 K5.2 75.56,46.36 71.12,41.91 | K8.2 38.73,66.67 41.27,64.13 41.27,55.24 K7.2 38.73,46.36 | 120.02,45.09 101.6,45.09 98.42,41.91 | 38.73,46.36 43.18,41.91 | v27.94,31.75 28,40.96 | 28,40.96 33.02,46.36 38.73,46.36 | C2.+ 8.38,54.48 10.16,52.7 10.16,45.09 11.43,43.81 25.15,43.81 28,40.96
  Bottom 1.778: 98.81,41.91 98.42,41.91 71.12,41.91 43.18,41.91 | v27.94,31.75 27.94,5.44 X2.2

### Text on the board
tNames: Bank 1 | 8 | 6 | 4 | 2 | 7 | 5 | 3 | 1 | A0 | A1 | A2 | SC | SCL | SDA | +5V | GND | 2016 ControlEverything.com | MCP23008 | ANSR8x0 | REV.A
